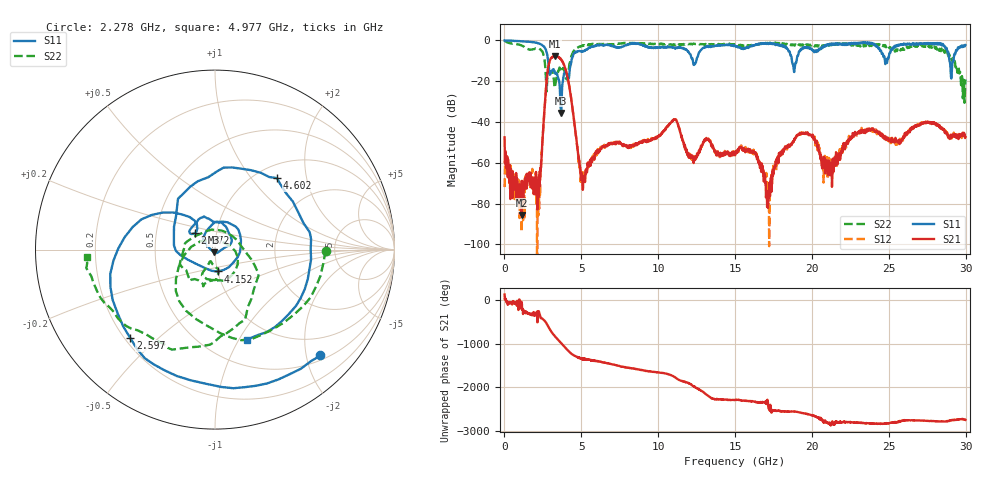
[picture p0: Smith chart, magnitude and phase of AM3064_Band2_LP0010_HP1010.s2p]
# Hz S DB R 50.0
!freq dBS11 angS11 dBS21 angS21 dBS12 angS12 dBS22 angS22
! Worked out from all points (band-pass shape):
!   1600 points, 10 MHz to 29.98 GHz, reference 50 ohm
!   highest |S21| = -7.63 dB at 3.271 GHz (marker M1); lowest = -85.6 dB at 1.116 GHz (marker M2)
!   |S21| within 3 dB of the highest: 2.921 GHz to 3.789 GHz (868.3 MHz wide, 25.9 % of centre)
!   lowest |S11| = -35.6 dB at 3.684 GHz (marker M3), VSWR 1.03, Z = 49.6 - j1.59 ohm
!   |S11| at or under -10 dB: 2.838 GHz to 4.356 GHz (1.518 GHz wide, 42.2 % of centre); 18.7 GHz to 19 GHz (297.4 MHz wide, 1.58 % of centre); 28.94 GHz to 29.2 GHz (255.9 MHz wide, 0.88 % of centre)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
!   |S22| runs from -30.6 to -0.2 dB; largest |S21 - S12| = 0.011
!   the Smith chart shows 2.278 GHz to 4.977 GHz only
!   S11 on the Smith chart (normalised r, x): 2.278 GHz: 0.59, -2.28; 2.597 GHz: 0.22, -0.41; 2.972 GHz: 0.78, +0.14; 4.152 GHz: 1.00, -0.25; 4.602 GHz: 1.23, +1.36; 4.977 GHz: 0.77, -1.08
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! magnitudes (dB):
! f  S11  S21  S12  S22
! 10 MHz  0.0  -47.5  -71.9  -0.2
! 1.116 GHz  -0.4  -85.6  -94.0  -2.5
! 2.278 GHz  -1.6  -71.8  -72.0  -4.2
! 2.597 GHz  -3.3  -34.4  -34.3  -9.1
! 2.972 GHz  -16.8  -9.5  -9.5  -15.2
! 3.271 GHz  -15.5  -7.6  -7.6  -23.2
! 3.684 GHz  -35.6  -9.4  -9.3  -13.4
! 4.152 GHz  -18.2  -19.9  -19.9  -16.7
! 4.602 GHz  -5.6  -43.8  -44.3  -4.3
! 4.977 GHz  -5.5  -68.5  -66.1  -2.9
! 5.015 GHz  -5.6  -66.5  -66.4  -2.9
! 10 GHz  -3.5  -47.2  -47.0  -1.8
! 15 GHz  -2.6  -56.3  -55.1  -1.9
! 16.26 GHz  -2.3  -55.0  -55.2  -2.4
! 17.16 GHz  -1.7  -79.4  -78.8  -1.4
! 17.99 GHz  -2.6  -54.6  -54.9  -1.5
! 19.99 GHz  -4.3  -47.1  -46.8  -2.1
! 21.19 GHz  -2.3  -62.4  -60.7  -1.8
! 22.8 GHz  -1.2  -44.9  -46.3  -2.6
! 25 GHz  -8.4  -49.1  -48.7  -3.0
! 28.56 GHz  -2.5  -43.9  -43.7  -4.7
! 29.98 GHz  -2.3  -47.3  -47.5  -19.2
